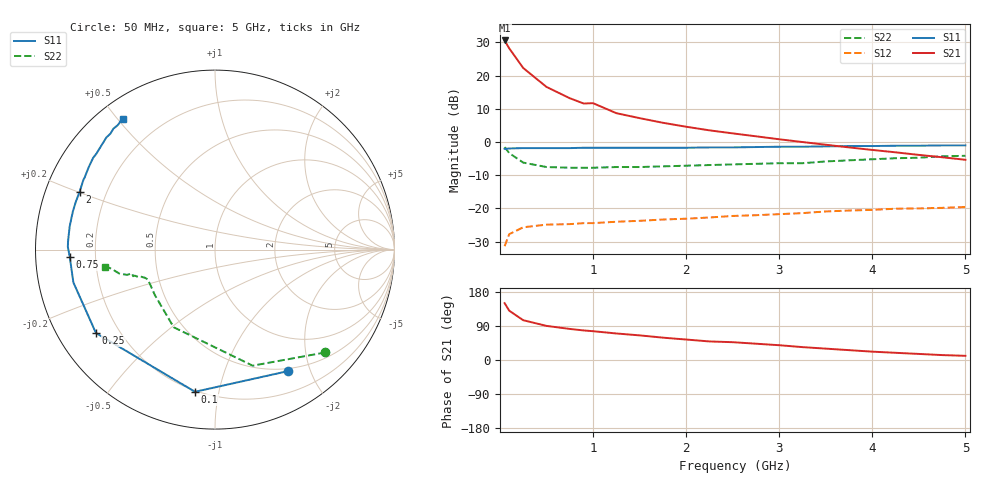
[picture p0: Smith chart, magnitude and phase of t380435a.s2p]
!AT-38043
!S-PARAMETERS at Vce=4.8V Ic=50mA. LAST UPDATED 01-06-98
# ghz s ma r 50
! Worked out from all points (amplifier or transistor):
!   23 points, 50 MHz to 5 GHz, reference 50 ohm
!   highest |S21| = 30.6 dB at 50 MHz (marker M1)
!   |S21| within 3 dB of that: start of sweep to 115.2 MHz
!   unconditionally stable (mu >= 1): 1.614 GHz to end of sweep
!   at 500 MHz: K = 0.39, MSG = 20.7 dB, |S12| = -24.9 dB
!   at 2.25 GHz: K = 1.21, MAG = 10.4 dB, |S12| = -22.7 dB
!   at 5 GHz: K = 1.29, MAG = 3.9 dB, |S12| = -19.6 dB
!   S11 on the Smith chart (normalised r, x): 50 MHz: 0.46, -1.67; 100 MHz: 0.19, -0.85; 250 MHz: 0.12, -0.31; 750 MHz: 0.11, -0.03; 2 GHz: 0.10, +0.20; 5 GHz: 0.07, +0.52
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0.05  0.79 -59.0  33.88 150.0  0.027 59.0  0.84 -43.0
0.1  0.8 -98.0  25.7 130.0  0.041 42.0  0.68 -72.0
0.25  0.81 -145.0  13.03 105.0  0.052 25.0  0.49 -118.0
0.5  0.81 -167.0  6.76 90.0  0.057 20.0  0.42 -143.0
0.75  0.81 -177.0  4.57 82.0  0.058 20.0  0.41 -152.0
0.9  0.82 179.0  3.8 78.0  0.06 21.0  0.41 -155.0
1  0.82 177.0  3.85 76.0  0.06 23.0  0.41 -156.0
1.25  0.82 171.0  2.72 70.0  0.063 25.0  0.42 -158.0
1.5  0.82 165.0  2.29 65.0  0.065 28.0  0.42 -158.0
1.75  0.82 161.0  1.95 59.0  0.068 30.0  0.43 -159.0
2  0.82 157.0  1.7 54.0  0.07 33.0  0.44 -160.0
2.25  0.83 152.0  1.5 49.0  0.073 36.0  0.45 -160.0
2.5  0.83 151.0  1.35 47.0  0.077 38.0  0.46 -161.0
2.75  0.84 147.0  1.22 43.0  0.079 42.0  0.47 -162.0
3  0.85 143.0  1.1 39.0  0.082 43.0  0.48 -162.0
3.25  0.85 141.0  1 34.0  0.085 44.0  0.48 -164.0
3.5  0.86 137.0  0.91 30.0  0.09 45.0  0.51 -164.0
4  0.87 132.0  0.76 22.0  0.095 46.0  0.55 -166.0
4.25  0.88 130.0  0.7 19.0  0.099 46.0  0.57 -168.0
4.5  0.88 128.0  0.64 16.0  0.1 46.0  0.58 -169.0
4.75  0.89 126.0  0.59 13.0  0.102 47.0  0.61 -171.0
5  0.89 125.0  0.54 11.0  0.105 47.0  0.62 -171.0
